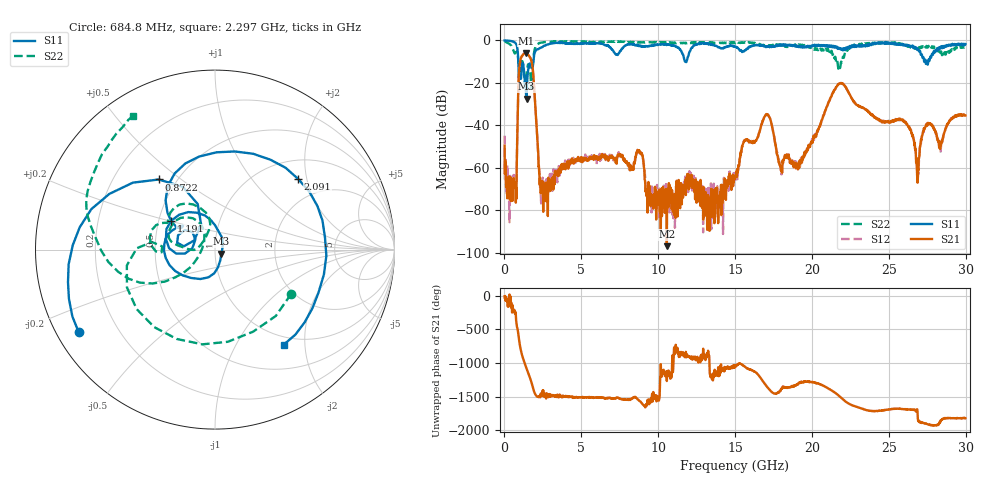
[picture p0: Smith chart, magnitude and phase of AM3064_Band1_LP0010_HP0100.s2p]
# Hz S DB R 50.0
!freq dBS11 angS11 dBS21 angS21 dBS12 angS12 dBS22 angS22
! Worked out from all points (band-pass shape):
!   1600 points, 10 MHz to 29.98 GHz, reference 50 ohm
!   highest |S21| = -5.87 dB at 1.397 GHz (marker M1); lowest = -97.0 dB at 10.56 GHz (marker M2)
!   |S21| within 3 dB of the highest: 1.052 GHz to 1.722 GHz (670.1 MHz wide, 48.3 % of centre)
!   lowest |S11| = -27.4 dB at 1.435 GHz (marker M3), VSWR 1.09, Z = 53.7 - j2.43 ohm
!   |S11| at or under -10 dB: 902 MHz to 1.877 GHz (975.5 MHz wide, 70.2 % of centre); 11.76 GHz to 11.84 GHz (87.97 MHz wide, 0.745 % of centre); 27.49047 GHz to 27.56431 GHz (73.84 MHz wide, 0.268 % of centre)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
!   |S22| runs from -22.9 to -0.3 dB; largest |S21 - S12| = 0.0065
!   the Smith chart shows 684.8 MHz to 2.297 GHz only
!   S11 on the Smith chart (normalised r, x): 684.8 MHz: 0.06, -0.28; 872.2 MHz: 0.40, +0.42; 1.191 GHz: 0.58, +0.21; 2.091 GHz: 1.43, +1.78; 2.297 GHz: 0.87, -1.60
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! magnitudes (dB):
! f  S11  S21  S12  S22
! 10 MHz  0.0  -49.6  -44.9  -0.3
! 684.8 MHz  -1.0  -66.8  -64.8  -6.2
! 872.2 MHz  -6.0  -31.2  -31.3  -7.2
! 1.191 GHz  -10.7  -6.9  -6.9  -10.4
! 1.397 GHz  -24.4  -5.9  -5.9  -18.7
! 1.435 GHz  -27.4  -6.0  -5.9  -16.4
! 1.791 GHz  -13.1  -10.8  -10.8  -17.5
! 2.091 GHz  -4.3  -41.2  -41.2  -2.1
! 2.297 GHz  -3.7  -68.1  -62.1  -1.2
! 5.015 GHz  -1.5  -56.2  -56.4  -0.8
! 8.782 GHz  -2.6  -52.7  -52.4  -0.9
! 10 GHz  -2.0  -72.4  -74.2  -0.9
! 10.56 GHz  -1.9  -97.0  -76.0  -1.2
! 15 GHz  -3.0  -65.0  -63.9  -1.4
! 17.03 GHz  -3.0  -34.8  -34.9  -2.6
! 17.97 GHz  -2.5  -59.8  -59.4  -2.1
! 19.99 GHz  -2.9  -48.2  -47.4  -3.5
! 21.85 GHz  -3.6  -20.2  -20.1  -12.5
! 25 GHz  -1.1  -38.3  -37.9  -1.1
! 26.85 GHz  -4.5  -65.4  -62.0  -3.1
! 27.49 GHz  -9.9  -40.3  -39.1  -3.2
! 29.98 GHz  -1.8  -35.4  -35.2  -3.1
